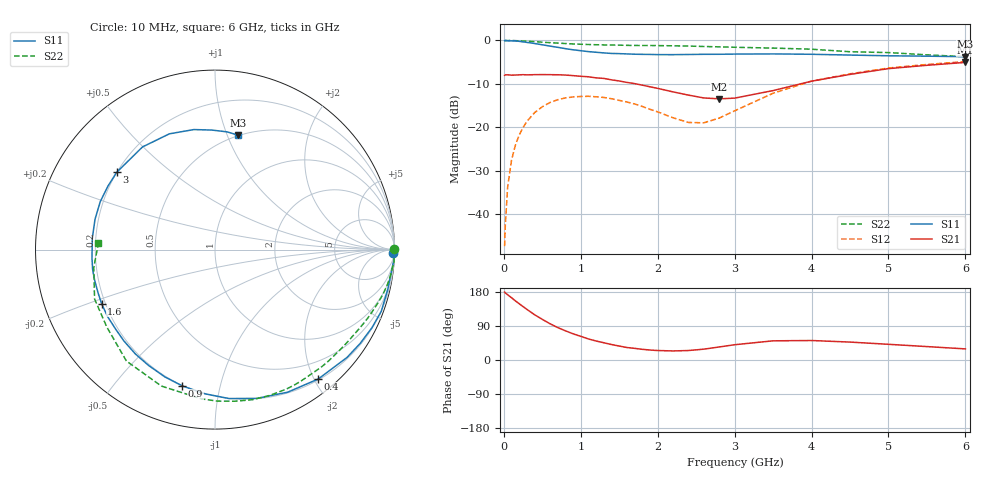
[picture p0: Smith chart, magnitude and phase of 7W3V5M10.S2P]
! Infineon Technologies  Discrete & RF Semiconductors
! BFS17W
! Si NPN RF Bipolar Junction Transistor in SOT323
! VCE = 3.5 V  IC = 0.1 mA
! Common Emitter S-Parameters:  August  1999
# GHz  S  MA  R  50
!  f  S11  S21  S12  S22
! GHz  MAG  ANG  MAG  ANG  MAG  ANG  MAG  ANG
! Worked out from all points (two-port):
!   36 points, 10 MHz to 6 GHz, reference 50 ohm
!   highest |S21| = -5.05 dB at 6 GHz (marker M1); lowest = -13.4 dB at 2.8 GHz (marker M2)
!   |S21| within 3 dB of the highest: start of sweep to 870.8 MHz; 4.422 GHz to end of sweep
!   lowest |S11| = -3.7 dB at 6 GHz (marker M3), VSWR 4.73, Z = 24.7 + j54.6 ohm
!   |S11| at or under -10 dB: nowhere
!   |S22| runs from -3.7 to 0.0 dB; largest |S21 - S12| = 0.4
!   S11 on the Smith chart (normalised r, x): 10 MHz: 27, -87; 400 MHz: 0.21, -2.06; 900 MHz: 0.20, -0.77; 1.6 GHz: 0.19, -0.22; 3 GHz: 0.20, +0.33; 6 GHz: 0.49, +1.09
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0.01  0.9936 -1.2  0.397 179.3  0.0043 88.7  0.9999 0.1
0.02  0.9999 -2.9  0.402 176.9  0.0078 91.6  0.9956 -0.8
0.05  0.9911 -6.7  0.402 172.0  0.0208 86.5  0.9986 -1.9
0.1  0.9878 -13.0  0.399 164.3  0.042 82.0  0.9999 -3.9
0.2  0.9768 -26.4  0.402 148.4  0.0818 73.1  0.9897 -7.7
0.3  0.9499 -39.2  0.402 133.6  0.1173 64.6  0.9806 -11.3
0.4  0.9223 -51.4  0.404 119.4  0.1478 56.9  0.9685 -14.9
0.6  0.8614 -74.2  0.404 95.7  0.1932 43.4  0.943 -21.2
0.9  0.7809 -103.5  0.394 69.1  0.2241 27.4  0.9117 -30.1
1.1  0.7439 -119.9  0.382 55.5  0.2278 19.1  0.8981 -35.8
1.3  0.7188 -134.9  0.366 45.5  0.221 12.6  0.8883 -41.7
1.6  0.6999 -154.5  0.329 32.9  0.1959 5.8  0.8784 -50.5
2.2  0.6866 174.7  0.256 23.9  0.1289 11.7  0.8678 -69.4
2.6  0.6929 157.3  0.218 28.6  0.1129 38.6  0.8521 -82.5
2.8  0.6934 149.3  0.213 34.4  0.1279 52.3  0.8441 -89.1
3  0.6968 141.8  0.217 40.3  0.155 61.1  0.8351 -95.2
3.5  0.7002 125.2  0.265 50.6  0.2471 66.2  0.8168 -111.5
4  0.6933 111.5  0.34 51.4  0.3404 60.7  0.7931 -128.5
4.5  0.6791 100.0  0.407 47.3  0.4132 52.9  0.7414 -144.3
5  0.6662 91.5  0.474 41.4  0.4817 45.2  0.7253 -157.7
5.5  0.6594 84.2  0.518 35.4  0.5295 37.8  0.683 -171.5
6  0.6507 78.7  0.559 29.3  0.5717 31.2  0.6504 176.6
